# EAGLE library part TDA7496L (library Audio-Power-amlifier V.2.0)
The TDA7496L is a stereo 2W+2W class AB power amplifier assembled in the @ Powerdip 14+3+3 package, specially designed for high quality sound, TV and Monitor applications. Features of the TDA7496L include linear volume control, Stand-by and mute functions.
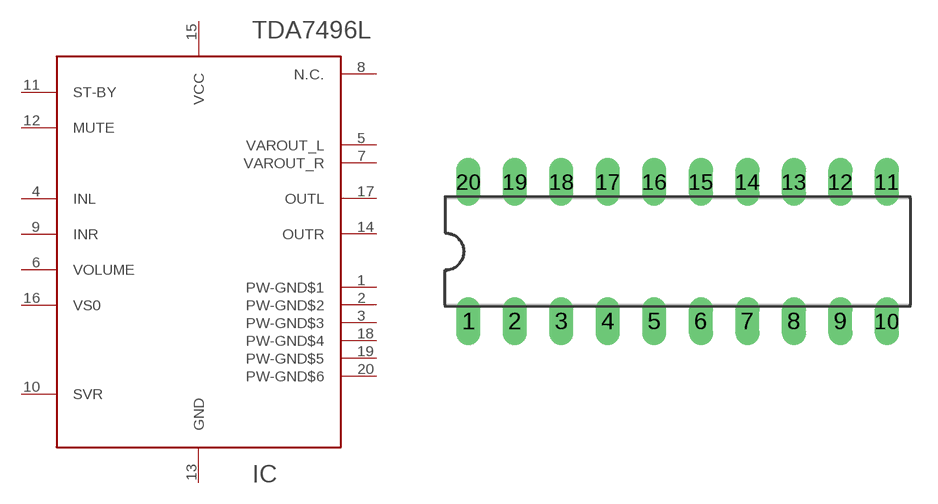
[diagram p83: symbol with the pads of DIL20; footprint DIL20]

Designator prefix IC

## TDA7496L  [DIL20]
1  PW-GND$1  sup
2  PW-GND$2  sup
3  PW-GND$3  sup
4  INL  in
5  VAROUT_L  out
6  VOLUME  in
7  VAROUT_R  out
8  N.C.  nc
9  INR  in
10  SVR  in
11  ST-BY  in
12  MUTE  in
13  GND  sup
14  OUTR  out
15  VCC  pwr
16  VS0  in
17  OUTL  out
18  PW-GND$4  sup
19  PW-GND$5  sup
20  PW-GND$6  sup

## Footprint DIL20 (pad centres in mm)
Dual In Line Package
drill 0.813 long: 1 -11.43,-3.81; 2 -8.89,-3.81; 3 -6.35,-3.81; 4 -3.81,-3.81; 5 -1.27,-3.81; 6 1.27,-3.81; 7 3.81,-3.81; 8 6.35,-3.81; 9 8.89,-3.81; 10 11.43,-3.81; 11 11.43,3.81; 12 8.89,3.81; 13 6.35,3.81; 14 3.81,3.81; 15 1.27,3.81; 16 -1.27,3.81; 17 -3.81,3.81; 18 -6.35,3.81; 19 -8.89,3.81; 20 -11.43,3.81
